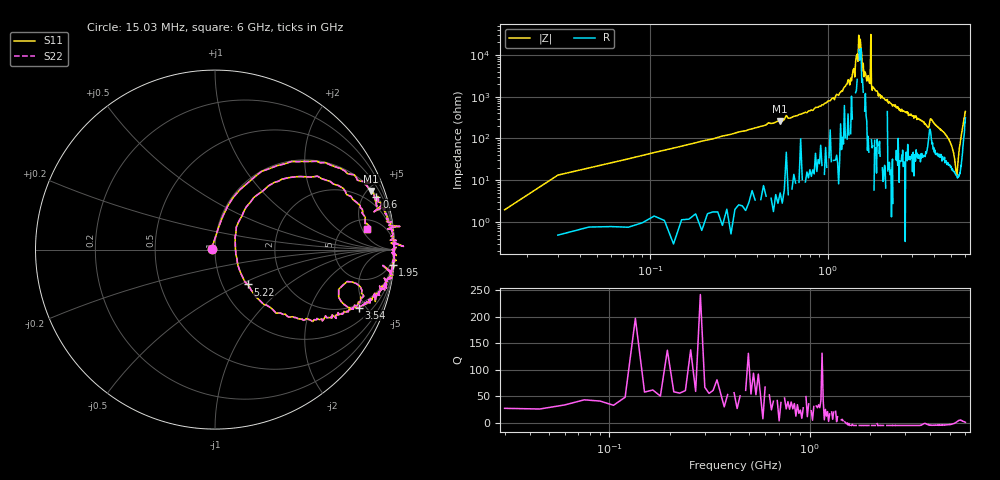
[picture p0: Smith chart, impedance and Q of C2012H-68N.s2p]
!	Network	Analyzer	HP8753E.07.74:	Oct	30	2002	Serial	No.	JP38451487
!	Hewlett-Packard
!	28	Aug	2009	10:28:00
!	Frequency	S11	S21	S12	S22
#	HZ	S	RI	R	50
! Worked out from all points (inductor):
!   400 points, 15.03 MHz to 6 GHz, reference 50 ohm
!   read as one part in series: L = 69.5 nH near 45.03 MHz
!   highest Q = 61.2 at 540 MHz (marker M1), where L = 77.8 nH
!   self-resonance near 1.515 GHz
!   S11 on the Smith chart (normalised r, x): 15.03 MHz: 0.96, +0.01; 600 MHz: 1.09, +6.08; 1.95 GHz: 2, -24; 3.54 GHz: 1.77, -4.48; 5.22 GHz: 1.31, -0.55; 6 GHz: 7.25, +6.31
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1.502992e7  -0.0186 0.00518  1.02 -0.00518  1.02 -0.00518  -0.0186 0.00518
3.002985e7  0.0217 0.129  0.978 -0.129  0.978 -0.129  0.0217 0.129
1.050295e8  0.182 0.371  0.818 -0.371  0.818 -0.371  0.182 0.371
5.400273e8  0.87 0.327  0.13 -0.327  0.13 -0.327  0.87 0.327
6.00027e8  0.899 0.294  0.101 -0.294  0.101 -0.294  0.899 0.294
1.020025e9  0.979 0.123  0.021 -0.123  0.021 -0.123  0.979 0.123
1.425023e9  1 0.0337  0.000184 -0.0337  0.000184 -0.0337  1 0.0337
1.500022e9  0.998 0.00299  0.00156 -0.00299  0.00156 -0.00299  0.998 0.00299
1.515022e9  0.987 0.000579  0.0132 -0.000579  0.0132 -0.000579  0.987 0.000579
1.725021e9  1 -0.0479  -0.00366 0.0479  -0.00366 0.0479  1 -0.0479
1.740021e9  0.996 -0.0469  0.00394 0.0469  0.00394 0.0469  0.996 -0.0469
1.755021e9  1 0.00311  -0.00091 -0.00311  -0.00091 -0.00311  1 0.00311
1.770021e9  0.995 -0.0518  0.00522 0.0518  0.00522 0.0518  0.995 -0.0518
1.785021e9  0.992 -0.0696  0.00784 0.0696  0.00784 0.0696  0.992 -0.0696
1.95002e9  0.99 -0.0839  0.0103 0.0839  0.0103 0.0839  0.99 -0.0839
2.01002e9  0.988 -0.0941  0.0116 0.0941  0.0116 0.0941  0.988 -0.0941
3.015015e9  0.917 -0.255  0.0835 0.255  0.0835 0.255  0.917 -0.255
3.540012e9  0.8 -0.323  0.2 0.323  0.2 0.323  0.8 -0.323
4.00501e9  0.791 -0.314  0.209 0.314  0.209 0.314  0.791 -0.314
5.010005e9  0.357 -0.353  0.643 0.353  0.643 0.353  0.357 -0.353
5.220004e9  0.182 -0.194  0.818 0.194  0.818 0.194  0.182 -0.194
6e9  0.847 0.117  0.153 -0.117  0.153 -0.117  0.847 0.117
